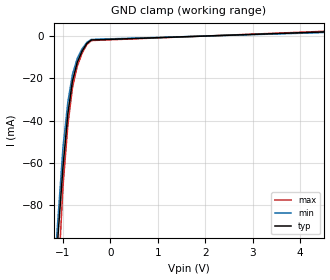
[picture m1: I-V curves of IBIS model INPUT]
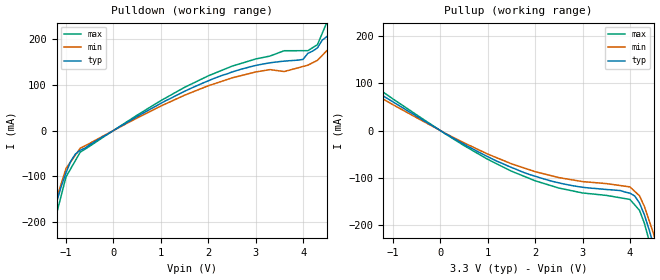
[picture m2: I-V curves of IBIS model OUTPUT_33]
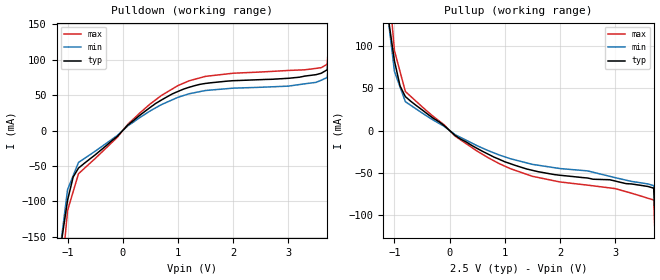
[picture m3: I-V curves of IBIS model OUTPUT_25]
|   PERICOM SEMICONDUCTOR CORP
|   IBIS Model of PI6C49X0210
|   Product Family: PI6C49Xxxx
|   TQFN (ZH) 32-pin Package
[IBIS Ver] 3.2
[Comment char] |_char
[File Name] pi6c49x0210.ibs
[File Rev] 2.0
[Source] File originated at Pericom Semiconductor Corp.
[Date] 09/06/13
[Disclaimer] (C) Copyright PERICOM Semiconductor Corporation
   All rights reserved
  Pericom Semiconductor Corporation hereby grants the user of
  this IBIS model a non-exclusive, nontransferable license to
  use this IBIS model under the following terms.
  This IBIS model is provided on an "AS IS" basis and Pericom
  makes absolutely no warranty with respect to the information
  contained herein. PERICOM DISCLAIMS AND CUSTOMER WAIVES ALL
  WARRANTIES, EXPRESSED OR IMPLIED, INCLUDING WARRANTIES OF
  MERCHANTABILITY OR FITNESS FOR A PARTICULAR PURPOSE. The
  entire risk as to quality and performance is with the customer.
  Accordingly, in no event shall the company be liable for any
  damages, whether in contract or tort, including any lost
  profits or other incidental, consequential, exemplary, or
  punitive damages arising out of the use or application of the
  IBIS model provided in this package. Further, Pericom reserves
  the right to make changes without notice to any product herein
  to improve reliability, function, or design. Pericom does not
  convey any license under patent rights or any other intellectual
  property rights, including those of third parties.
  The user is granted this license only to use the IBIS model
  and is not granted rights to sell, load, rent, lease or license
  the IBIS model in whole or in part, or in modified form to anyone
  other than user. User may modify the IBIS model to suit its specific
  application but rights to derivative works and such modifications
  shall belong to Pericom.
  Pericom is not obligated to provide maintenance or support
  for the licensed IBIS model.
  Contact Pericom at ATTN: APPLICATION ENGINEERING / IBIS MODELS
  3545 North First Street, San Jose, CA 95134
[Component] pi6c49x0210
[Manufacturer] Pericom Semiconductor Corp.
[Package]
| variable   typ   min  max
R_pkg   0.52715ohm  0.474435	0.579865
L_pkg   1.17050nH   1.01345nH	1.22755nH
C_pkg   0.29280pF   0.26352pF	0.32208pF
[Pin]   Signal_Name   Model_Name   R_pin   L_pin   C_pin
1   CLK0   OUTPUT   0.05379   1.258nH   0.2294pF
2   VDDO   POWER   0.05379   1.458nH   0.2294pF
3   CLK1   OUTPUT   0.05379   1.258nH   0.2294pF
4   GNDO   GND   0.05379   1.458nH   0.2294pF
5   CLK2   OUTPUT   0.05379   1.258nH   0.2294pF
6   VDDO   POWER   0.05379   1.458nH   0.2294pF
7   CLK3   OUTPUT   0.05379   1.258nH   0.2294pF
8   CLK4   OUTPUT   0.05379   1.258nH   0.2294pF
9   GNDO   GND   0.05379   1.458nH   0.2294pF
10   VDD   POWER   0.05379   1.458nH   0.2294pF
11   XIN   INPUT   0.05164   1.483nH   0.3562pF
12   XOUT   OUTPUT   0.05379   1.258nH   0.2294pF
13   IN0   INPUT   0.05164   1.483nH   0.3562pF
14   IN0#   INPUT   0.05164   1.483nH   0.3562pF
15   GND   GND   0.05379   1.458nH   0.2294pF
16   GNDO   GND   0.05379   1.458nH   0.2294pF
17   CLK5   OUTPUT   0.05379   1.258nH   0.2294pF
18   CLK6   OUTPUT   0.05379   1.258nH   0.2294pF
19   VDDO   GND   0.05379   1.458nH   0.2294pF
20   CLK7   OUTPUT   0.05379   1.258nH   0.2294pF
21   GNDO   GND   0.05379   1.458nH   0.2294pF
22   CLK8   OUTPUT   0.05379   1.258nH   0.2294pF
23   VDDO   GND   0.05379   1.458nH   0.2294pF
24   CLK9   OUTPUT   0.05379   1.258nH   0.2294pF
25   GNDO   GND   0.05379   1.458nH   0.2294pF
26   GND   GND   0.05379   1.458nH   0.2294pF
27   IN1#   INPUT   0.05164   1.483nH   0.3562pF
28   IN1   INPUT   0.05164   1.483nH   0.3562pF
29   IN_SEL1   INPUT   0.05164   1.483nH   0.3562pF
30   IN_SEL0   INPUT   0.05164   1.483nH   0.3562pF
31   ENABLE   INPUT   0.05164   1.483nH   0.3562pF
32   GNDO   GND   0.05379   1.458nH   0.2294pF
| OUTPUT model selection
[Model Selector]   OUTPUT
OUTPUT_33   3.3 volt VDD
OUTPUT_25   2.5 volt VDD
OUTPUT_18   1.8 volt VDD
OUTPUT_15   1.5 volt VDD
| Models and submodels in the file (5): INPUT (Input), OUTPUT_33 (Output), OUTPUT_25 (Output), OUTPUT_18 (Output), OUTPUT_15 (Output)
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|   Model INPUT
[Model] INPUT
Model_type Input
Vinl = 400mV
Vinh = 3.0V
| variable   typ   min   max
C_comp   2.000pF   1.8pF	2.2pF
[Voltage Range]   3.300V   3.0	 3.6
[POWER Clamp Reference]   2.500V   NA   NA
[GND Clamp Reference]   0.000V   0	 0
[Pullup Reference]   3.300V   3.3	 3.3
[Pulldown Reference]   0.000V   NA   NA
[Temperature Range]   25.00   85.00   -45.000
[GND Clamp]
| Voltage   I(typ)   I(min)   I(max)
-2.501V   -689.3mA   -585.9mA   -792.7mA
-1.202V   -128.3mA   NA         NA
-1.1V     -92.86mA   NA         NA
-999.3mV  -61.6mA    -52.36mA   -70.84mA
-898.2mV  -36.82mA   -31.3mA    -42.34mA
-802mV    -21.38mA   -18.17mA   -24.59mA
-700.9mV  -12.48mA   -10.61mA   -14.35mA
-599.7mV  -7.15mA    -6.077mA   -8.223mA
-498.6mV  -3.5mA     -2.975mA   -4.025mA
-402.7mV  -1.81mA    -1.538mA   -2.082mA
4.999V    2.38mA     2.023mA    2.737mA
[POWER Clamp]   |Note: Vtable = Vcc - Voutput
| Voltage   I(typ)   I(min)   I(max)
-2.501V   0A         0A         0A
0V        0A         0A         0A
|   Model OUTPUT_33
[Model] OUTPUT_33
Model_type Output
Vref = 0.0000V
Rref = 500ohms
Vmeas = 1.650V
| variable   typ   min   max
C_comp   2.000pF   1.8pF	2.2pF
[Voltage Range]   3.300V   3.0	 3.6
[POWER Clamp Reference]   3.300V   NA   NA
[GND Clamp Reference]   0.000V   0	 0
[Pullup Reference]   3.300V   3.0	 3.6
[Pulldown Reference]   0.000V   NA   NA
[Temperature Range]   25.00   85.00   -45.000
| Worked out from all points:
|   slope of the pulldown table from 0 to 0.495 V, typ, clamps not added: 16.3 ohm
|   slope of the pullup table from 0 to 0.495 V, typ, clamps not added: 17.3 ohm
[Pulldown]
| Voltage   I(typ)   I(min)   I(max)
-3.3V     -970.1mA   -873.1mA   -1.067A
-1.5V     -275.4mA   -247.9mA   -302.9mA
-1.399V   -233.1mA   NA         NA
-1.303V   -195.7mA   NA         NA
-999.7mV  -92.08mA   -82.87mA   -101.3mA
-701.1mV  -43.09mA   -38.78mA   -47.4mA
2.001V    108.7mA    97.87mA    119.6mA
4.099V    168.7mA    142.8mA    174.5mA
4.301V    180.6mA    153.5mA    187.7mA
4.499V    205.3mA    174.5mA    236.1mA
5.101V    265.9mA    NA         NA
6.602V    864.3mA    734.7mA    994mA
[Pullup]   |Note: Vtable = Vcc - Voutput
| Voltage   I(typ)   I(min)   I(max)
-3.3V     222.2mA    200mA      244.4mA
-2.901V   201.6mA    NA         NA
-2.8V     194.9mA    NA         NA
-1.5V     92.51mA    83.26mA    101.8mA
99.58mV   -6.14mA    -5.526mA   -6.754mA
1.202V    -65.12mA   NA         NA
2.501V    -110.4mA   -99.4mA    -121.5mA
3.998V    -132.2mA   -119mA     -145.4mA
4.2V      -153.2mA   -137.9mA   -168.5mA
4.402V    -209.4mA   NA         NA
4.499V    -243mA     -218.7mA   -267.3mA
6.603V    -1.056A    -950.8mA   -1.162A
[Ramp]
| variable   typ   min   max
dV/dt_r   2.0V/941.0p   2.0V/1041.0p   2.0V/841.0p
dV/dt_f   2.0V/806.0p   2.0V/1006.0p   2.0V/706.0p
R_load = 500ohms
|   Model OUTPUT_25
[Model] OUTPUT_25
Model_type Output
Vref = 0.0000V
Rref = 500ohms
Vmeas = 1.250V
| variable   typ   min   max
C_comp   2.000pF   1.8pF	2.2pF
[Voltage Range]   2.500V   2.375	 2.625
[POWER Clamp Reference]   2.500V   NA   NA
[GND Clamp Reference]   0.000V   0	 0
[Pullup Reference]   2.500V   2.375	 2.625
[Pulldown Reference]   0.000V   NA   NA
[Temperature Range]   25.00   85.00   -45.000
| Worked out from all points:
|   slope of the pulldown table from 0 to 0.375 V, typ, clamps not added: 14.8 ohm
|   slope of the pullup table from 0 to 0.375 V, typ, clamps not added: 22.6 ohm
[Pulldown]
| Voltage   I(typ)   I(min)  I(max)
-2.501V   -1.346A    -1.144A    -1.548A
-1.1V     -151.1mA   NA         NA
-999.3mV  -97.83mA   -83.16mA   -112.5mA
-898.2mV  -65.44mA   NA         NA
-802mV    -52.94mA   -45mA      -60.88mA
301.5mV   21.02mA    17.87mA    24.17mA
999.4mV   55.02mA    46.77mA    63.27mA
1.5V      66.36mA    56.41mA    76.31mA
3.502V    78.7mA     67.85mA    87.55mA
3.708V    85.7mA     74.84mA    93.55mA
3.801V    230.1mA    NA         NA
4.999V    1.25A      1.063A     1.438A
[Pullup]   |Note: Vtable = Vcc - Voutput
| Voltage   I(typ)   I(min)   I(max)
-2.501V   1.292A     1.098A     1.485A
-1.1V     128.3mA    NA         NA
-999.4mV  82.22mA    69.89mA    94.55mA
-898.2mV  52.83mA    NA         NA
-802mV    40.18mA    34.15mA    46.21mA
99.44mV   -5.76mA    -4.896mA   -6.624mA
898.2mV   -34.05mA   -28.94mA   -39.16mA
1.601V    -48.71mA   NA         NA
3.002V    -59.8mA    -55.83mA   -68.77mA
3.699V    -68.29mA   -65.3mA    -82.28mA
3.801V    -203.5mA   NA         NA
4.999V    -1.244A    -1.058A    -1.431A
[Ramp]
| variable   typ   min   max
dV/dt_r   2.0V/941.0p   2.0V/1041.0p   2.0V/841.0p
dV/dt_f   2.0V/806.0p   2.0V/1006.0p   2.0V/706.0p
R_load = 500ohms
